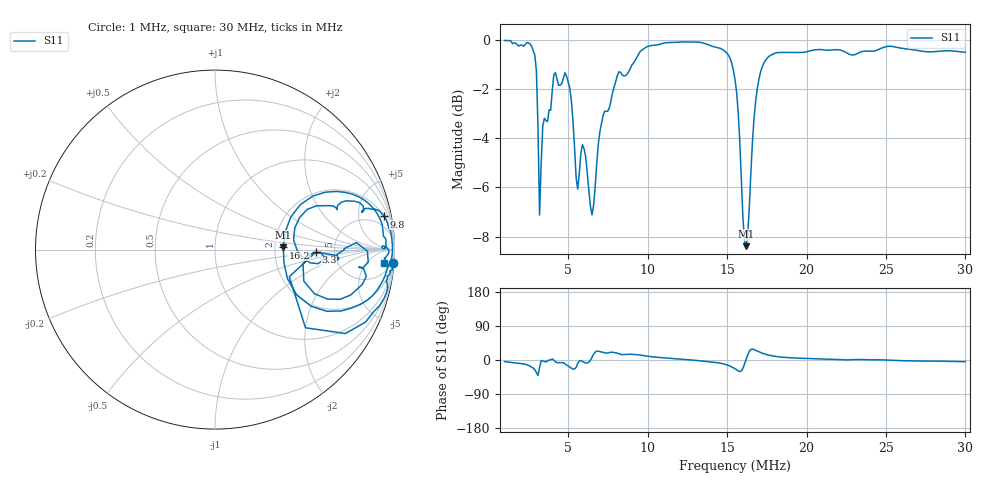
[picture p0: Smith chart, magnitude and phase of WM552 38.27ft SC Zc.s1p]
!Created via Zplots "Save as S1P" button
!Original data file:  $remote$.s1p
!Transmission line transform:  None
# MHZ S MA R 50
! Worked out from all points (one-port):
!   291 points, 1 MHz to 30 MHz, reference 50 ohm
!   lowest |S11| = -8.4 dB at 16.2 MHz (marker M1), VSWR 2.23, Z = 111 + j3.19 ohm
!   |S11| at or under -10 dB: nowhere
!   S11 on the Smith chart (normalised r, x): 1 MHz: 2, -27; 3.3 MHz: 3.55, -0.16; 9.8 MHz: 2, +10; 16.2 MHz: 2.23, +0.06; 30 MHz: 13, -16
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1  0.9956 -4.2
2.5  0.9845 -14.3
3  0.8642 -32.8
3.1  0.6661 -40.8
3.2  0.4406 -20.0
3.3  0.5611 -1.5
4.1  0.8491 -0.6
4.7  0.8357 -7.4
5.3  0.6855 -23.7
5.5  0.5248 -19.5
5.7  0.5353 -2.6
5.9  0.6119 -4.1
6.5  0.4408 7.1
6.9  0.6155 23.4
8.3  0.8578 14.8
9.8  0.9599 11.1
11.9  0.9872 2.8
14.7  0.9551 -9.6
15.5  0.8296 -23.0
15.8  0.6215 -30.5
16.2  0.3809 1.8
16.5  0.5373 27.8
16.8  0.7494 25.6
17.6  0.922 13.1
19.2  0.9411 5.4
22.8  0.9313 0.6
26.4  0.9563 -2.2
30  0.9421 -4.4
